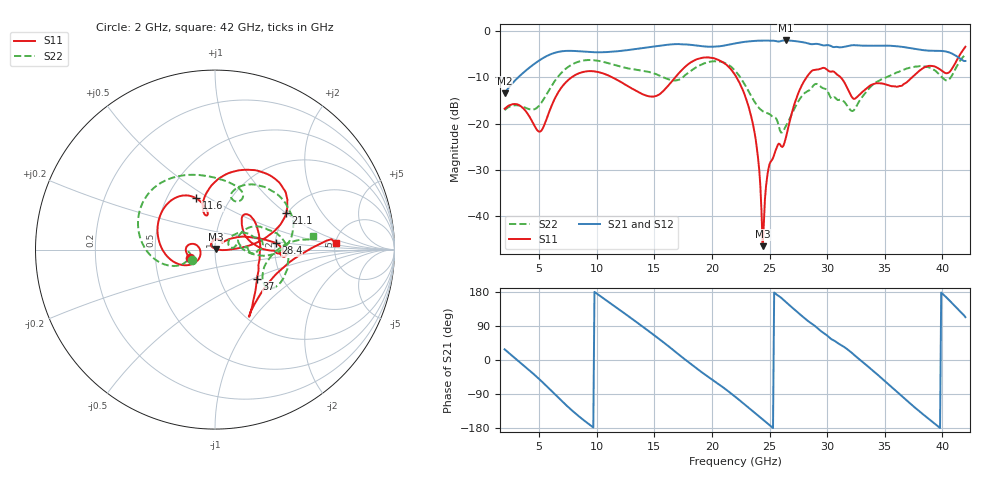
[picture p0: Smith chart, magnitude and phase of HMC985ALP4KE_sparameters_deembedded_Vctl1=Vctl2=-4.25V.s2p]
!s2p File: Measurements: S11, S21, S12, S22
# GHz S dB R 50.0
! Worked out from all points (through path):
!   401 points, 2 GHz to 42 GHz, reference 50 ohm
!   highest |S21| = -2.07 dB at 26.4 GHz (marker M1); lowest = -13.4 dB at 2 GHz (marker M2)
!   lowest |S11| = -46.4 dB at 24.4 GHz (marker M3), VSWR 1.01, Z = 50.3 + j0.369 ohm
!   |S11| at or under -10 dB: start of sweep to 7.828 GHz; 22.13 GHz to 28.22 GHz (6.092 GHz wide, 24.2 % of centre); 31.16 GHz to 37.39 GHz (6.224 GHz wide, 18.2 % of centre)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
!   |S22| runs from -21.9 to -5.2 dB; largest |S21 - S12| = 0.00071
!   S11 on the Smith chart (normalised r, x): 2 GHz: 0.76, -0.07; 11.6 GHz: 0.70, +0.44; 21.1 GHz: 1.98, +1.00; 28.4 GHz: 2.01, +0.17; 37 GHz: 1.50, -0.53; 42 GHz: 5.05, +0.66
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2  -16.80 -161.9  -13.45 28.1  -13.46 28.1  -17.10 -155.8
5  -21.73 -173.9  -6.39 -50.3  -6.40 -50.3  -16.11 -160.5
6.3  -14.90 -151.0  -4.78 -88.5  -4.78 -88.5  -11.01 -162.1
8.7  -8.94 150.0  -4.45 -154.8  -4.45 -154.8  -6.46 150.9
11.6  -10.35 110.1  -4.45 140.6  -4.45 140.6  -7.39 103.1
13.6  -13.19 101.5  -3.84 96.7  -3.85 96.7  -8.45 75.3
15.4  -13.75 106.5  -3.24 55.8  -3.24 55.8  -9.58 62.0
17.9  -7.26 79.7  -2.96 -4.4  -2.96 -4.4  -9.12 72.0
21.1  -7.03 27.0  -3.15 -75.2  -3.15 -75.2  -6.91 15.4
22  -9.47 16.6  -2.71 -96.5  -2.72 -96.5  -8.56 0.0
23.6  -20.66 0.9  -2.19 -136.3  -2.19 -136.3  -14.90 -3.9
24.4  -46.41 50.1  -2.10 -156.4  -2.10 -156.4  -17.32 8.0
25  -28.70 128.6  -2.12 -171.7  -2.12 -171.7  -17.96 11.8
26.4  -23.19 41.6  -2.07 153.5  -2.07 153.5  -20.65 33.6
28.4  -9.37 6.1  -2.75 101.4  -2.75 101.4  -12.88 17.7
28.7  -8.57 1.2  -2.88 95.2  -2.88 95.2  -12.18 15.8
32.4  -14.65 29.7  -3.10 11.9  -3.09 11.8  -16.85 26.2
33.9  -11.57 48.3  -3.21 -26.3  -3.21 -26.3  -11.76 30.2
35.4  -11.76 18.0  -3.21 -66.3  -3.21 -66.3  -9.73 18.9
37  -10.89 -34.8  -3.63 -109.4  -3.63 -109.4  -8.07 4.2
39.8  -8.33 -56.4  -4.32 -179.4  -4.32 -179.4  -9.55 -34.9
42  -3.42 3.0  -6.50 113.0  -6.50 113.0  -5.17 7.8
